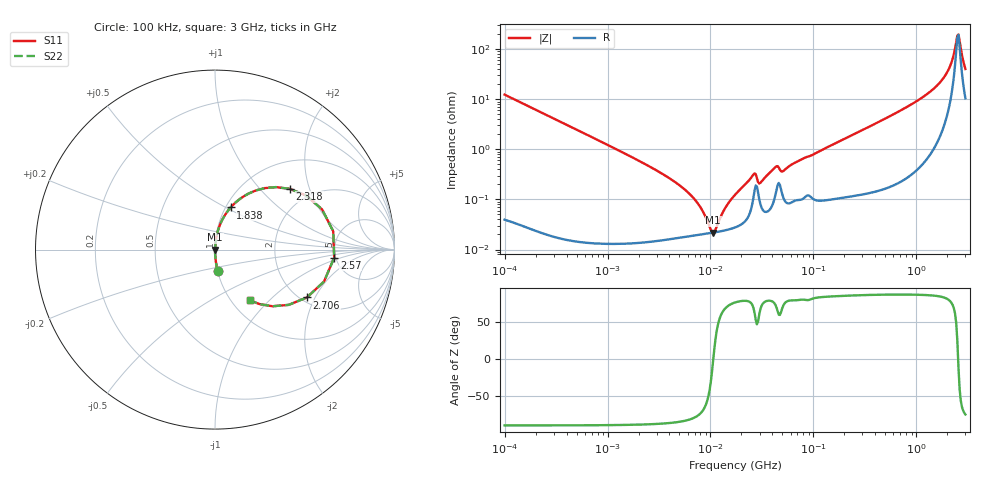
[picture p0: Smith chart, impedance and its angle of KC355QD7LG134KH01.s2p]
!Murata Part Number: KC355QD7LG134KH01
!These Parameters are Measured in Series Mode Connection
!Data Generated on Jun 19, 2026
!  o--ll--o
!Port1  Port2
!  o------o
!Operation Temp=25[degC], DC Bias Voltage=0[V]
!Freq. Start=100[kHz] Stop=3[GHz] 401[Steps]
# Hz S RI R 50
!Freq.(Hz) S11(Real) S11(Imag) S21(Real) S21(Imag) S12(Real) S12(Imag) S22(Real) S22(Imag)
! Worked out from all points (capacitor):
!   401 points, 100 kHz to 3 GHz, reference 50 ohm
!   read as one part in series: C = 129 nF near 105.3 kHz
!   lowest |Z| = 21.7 mohm at 10.61 MHz (marker M1)
!   series resonance near 10.65 MHz, so ESL is about 1.7 nH
!   S11 on the Smith chart (normalised r, x): 100 kHz: 1.00, -0.25; 1.838 GHz: 1.06, +0.53; 2.318 GHz: 1.57, +1.49; 2.57 GHz: 4.86, -0.78; 2.706 GHz: 2.16, -1.73; 3 GHz: 1.21, -0.78
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100000  0.0155 -0.1218  0.9845 0.1218  0.9845 0.1218  0.0155 -0.1218
562235  0.000623 -0.022  0.9994 0.022  0.9994 0.022  0.000623 -0.022
3161081  0.000162 -0.00355  0.9998 0.00355  0.9998 0.00355  0.000162 -0.00355
6674626  0.000189 -0.00111  0.9998 0.00111  0.9998 0.00111  0.000189 -0.00111
7994228  0.000199 -0.000668  0.9998 0.000668  0.9998 0.000668  0.000199 -0.000668
1.061445e7  0.000217 -8e-06  0.9998 8e-06  0.9998 8e-06  0.000217 -8e-06
1.409348e7  0.000244 0.000661  0.9998 -0.000661  0.9998 -0.000661  0.000244 0.000661
1.77727e7  0.000282 0.00128  0.9997 -0.00128  0.9997 -0.00128  0.000282 0.00128
2.616047e7  0.00109 0.00294  0.9989 -0.00294  0.9989 -0.00294  0.00109 0.00294
3.053531e7  0.000816 0.00198  0.9992 -0.00198  0.9992 -0.00198  0.000816 0.00198
4.268829e7  0.00122 0.00423  0.9988 -0.00423  0.9988 -0.00423  0.00122 0.00423
5.112795e7  0.00109 0.00354  0.9989 -0.00354  0.9989 -0.00354  0.00109 0.00354
9.738194e7  0.00111 0.00761  0.9989 -0.00761  0.9989 -0.00761  0.00111 0.00761
5.475153e8  0.00379 0.0451  0.9962 -0.0451  0.9962 -0.0451  0.00379 0.0451
1.186261e9  0.018 0.1115  0.982 -0.1115  0.982 -0.1115  0.018 0.1115
1.838476e9  0.0871 0.2347  0.9129 -0.2347  0.9129 -0.2347  0.0871 0.2347
2.091327e9  0.1887 0.313  0.8113 -0.313  0.8113 -0.313  0.1887 0.313
2.318426e9  0.4175 0.3384  0.5825 -0.3384  0.5825 -0.3384  0.4175 0.3384
2.441062e9  0.5964 0.2244  0.4036 -0.2244  0.4036 -0.2244  0.5964 0.2244
2.570185e9  0.6644 -0.0445  0.3356 0.0445  0.3356 0.0445  0.6644 -0.0445
2.706139e9  0.5125 -0.2664  0.4875 0.2664  0.4875 0.2664  0.5125 -0.2664
3e9  0.1947 -0.2835  0.8053 0.2835  0.8053 0.2835  0.1947 -0.2835
